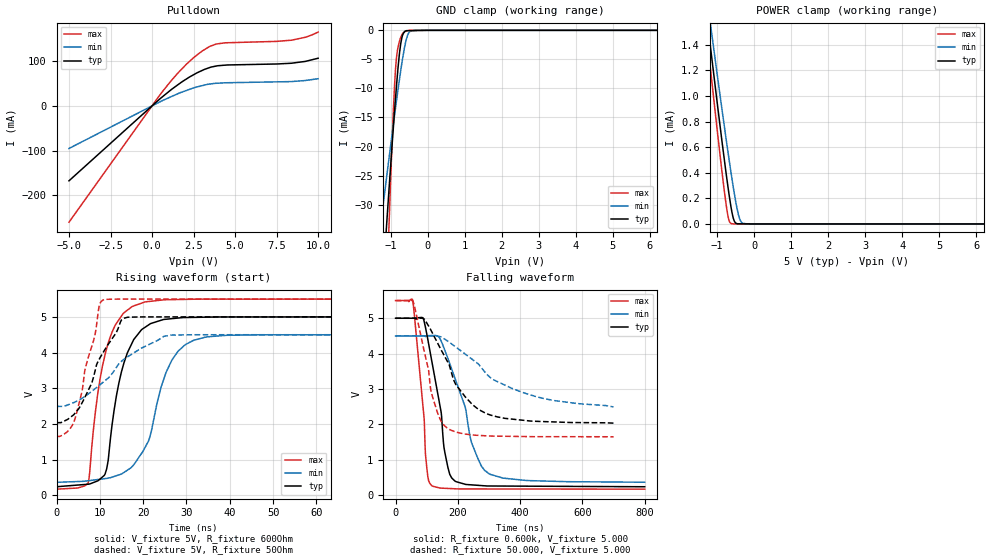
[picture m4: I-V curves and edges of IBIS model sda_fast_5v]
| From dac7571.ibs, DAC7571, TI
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|   SDA_5V IO OPEN DRAIN MODEL
|   5.0V fast mode, freq-3.4M,Rload=600ohm,  Cload = 15pF
[Model]   sda_fast_5v
Model_type   I/O_open_drain
Polarity   Non-Inverting
Enable   Active-Low
Vinl = 1.5
Vinh = 3.5
Vmeas = 2.5
Vref = 5.0
Cref = 15pF
Rref = 600
|   typ   min   max
|   (nom PVT)   (Fast PVT)   (Slow PVT)
|Average
C_comp   5.040e-12   2.855e-12   5.061e-12
|ON state : BUFFER OUTPUT TURNED LOW
|C_comp   6.129e-11   2.855e-11   1.162e-10
|OFF state : BUFFER IN HIGH IMPEDANCE STATE
|C_comp   5.061e-12   5.094e-12   5.040e-12
|Where nom PVT is NOM Process, 5.0V,25C
|   Fast PVT is Strong Process, 5.5V, -40C
|   Slow PVT is Weak Process, 4.5V, 105C
[Model spec]
|   typ   min   max
Vinl   1.5   1.35   1.65
Vinh   3.5   3.15   3.85
[Voltage Range]   5   4.5   5.5
|Junction temperature
[Temperature Range]   25   105   -40
[Pullup Reference]   5   4.5   5.5
[Pulldown Reference]   0   0   0
[Power Clamp Reference]   5   4.5   5.5
[GND Clamp Reference]   0   0   0
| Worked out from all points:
|   slope of the pulldown table from 0 to 0.75 V, typ, clamps not added: 31.1 ohm
|   GND clamp passes 1 mA (typ) near -0.68 V on its own axis
|   POWER clamp passes 1 mA (typ) near -1.02 V on its own axis
|   falling waveform, R_fixture 0.600k, V_fixture 5.000: 20-80 % time 47.7ns typ, 81.4ns min, 28.1ns max; typ from 5 V to 0.238 V
|   rising waveform, V_fixture 5V, R_fixture 600Ohm: 20-80 % time 4.46ns typ, 6.46ns min, 4.34ns max; typ from 0.238 V to 5 V
|   falling waveform, R_fixture 50.000, V_fixture 5.000: 20-80 % time 111ns typ, 204ns min, 55.6ns max; typ from 5 V to 2.04 V
|   rising waveform, V_fixture 5V, R_fixture 50Ohm: 20-80 % time 6.88ns typ, 11.3ns min, 4.33ns max; typ from 2.03 V to 5 V
[Pulldown]
|   Voltage   I(typ)   I(min)   I(max)
-5V       -167.6mA   -95.21mA   -260.1mA
632mV     20.56mA    11.88mA    32.24mA
1.567V    47.51mA    27.48mA    73.88mA
2.073V    60.23mA    34.53mA    93.27mA
3.03V     79.48mA    45.34mA    123mA
3.475V    85.81mA    48.85mA    133mA
3.866V    89.13mA    50.56mA    138.4mA
4.41V     91.14mA    51.64mA    141.1mA
7.49V     93.71mA    53.75mA    144.3mA
8.398V    95.44mA    54.36mA    146.9mA
9.239V    99.6mA     56.83mA    153.6mA
10V       106.6mA    60.8mA     165.1mA
[GND Clamp]
|   Voltage   I(typ)   I(min)   I(max)
-5V       -412.1mA   -229.4mA   -786.8mA
-1.266V   -48.89mA   -33.49mA   -75.73mA
-1.101V   -33mA      -25.04mA   -44.62mA
-1.04V    -27.31mA   -21.99mA   -33.44mA
-924.5mV  -16.82mA   -16.27mA   -14.04mA
-886mV    -13.47mA   -14.41mA   -8.932mA
-847.5mV  -10.29mA   -12.56mA   -5.324mA
-725mV    -2.321mA   -6.967mA   -1.233mA
-575mV    -62.02uA   -1.604mA   -142.6uA
-495.5mV  -53.37uA   -326.8uA   -12.8uA
-324.5mV  -34.76uA   -2.562uA   -8.377uA
10V       0A         0A         0A
[POWER Clamp]
|   Voltage   I(typ)   I(min)   I(max)
-5V       10.92mA    10.1mA     11.74mA
-1.335V   1.762mA    1.9mA      1.632mA
-1.265V   1.591mA    1.747mA    1.443mA
-1.238V   1.526mA    1.688mA    1.371mA
-1.15V    1.313mA    1.498mA    1.136mA
-748.5mV  378.2uA    647.3uA    135.5uA
-688mV    251.5uA    526.5uA    38.06uA
-622mV    128.1uA    396.8uA    2.687uA
-535mV    22.14uA    238.1uA    46.65nA
-428mV    1.278uA    76.93uA    37.34nA
-306.5mV  910.7nA    4.902uA    26.77nA
10V       0A         0A         0A
[Ramp]
R_load = 600
|   typ   min   max
dV/dt_r   2.85718/4.40572e-09   2.48289/6.38671e-09   3.19799/4.32733e-09
dV/dt_f   2.78474/4.60403e-08   0.852531/3.54328e-08   3.19353/2.80374e-08
[Falling Waveform]
R_fixture = 0.600k
V_fixture = 5.000
V_fixture_min = 4.500
V_fixture_max = 5.500
|  time   V(typ)   V(min)   V(max)
0s        5V         4.5V       5.5V
55.1ns    5V         4.5V       5.502V
91.66ns   4.916V     4.5V       2.169V
100.2ns   4.557V     4.498V     786mV
116.1ns   3.799V     4.511V     271.3mV
159.1ns   1.17V      4.073V     194.2mV
192ns     393.3mV    3.272V     181mV
245.1ns   290.7mV    1.458V     176.7mV
302.4ns   259.8mV    597.8mV    176mV
800ns     238.2mV    366mV      170mV
[Rising Waveform]
V_fixture = 5V
V_fixture_min = 4.5V
V_fixture_max = 5.5V
R_fixture = 600Ohm
|   Time   V(typ)   V(min)   V(max)
0s        238mV      361.8mV    170mV
7.308ns   308.7mV    406.2mV    351.7mV
9.414ns   397.8mV    438.6mV    2.753V
11.17ns   586.8mV    465.6mV    3.922V
14.4ns    3.148V     570.1mV    4.919V
17.53ns   4.29V      811.7mV    5.295V
21.26ns   4.775V     1.525V     5.432V
26.6ns    4.95V      3.781V     5.484V
31.64ns   4.987V     4.343V     5.495V
100ns     5V         4.5V       5.5V
[Falling Waveform]
R_fixture = 50.000
V_fixture = 5.000
V_fixture_min = 4.500
V_fixture_max = 5.500
|  time   V(typ)   V(min)   V(max)
0s        5V         4.5V       5.5V
56.25ns   5V         4.5V       5.473V
105.7ns   4.786V     4.501V     3.543V
117.4ns   4.597V     4.501V     2.819V
144.6ns   4.135V     4.477V     2.119V
173.3ns   3.654V     4.319V     1.857V
223ns     2.786V     3.991V     1.727V
300.8ns   2.276V     3.35V      1.673V
461.9ns   2.084V     2.762V     1.653V
700ns     2.036V     2.493V     1.65V
[Rising Waveform]
V_fixture = 5V
V_fixture_min = 4.5V
V_fixture_max = 5.5V
R_fixture = 50Ohm
|   Time   V(typ)   V(min)   V(max)
0s        2.033V     2.492V     1.65V
4.178ns   2.286V     2.606V     2.114V
5.884ns   2.588V     2.717V     2.906V
6.654ns   2.772V     2.778V     3.569V
8.845ns   3.46V      2.981V     4.474V
9.878ns   3.819V     3.083V     5.318V
10.76ns   4.001V     3.169V     5.474V
15.55ns   4.963V     3.812V     5.5V
26.44ns   5V         4.489V     5.5V
100ns     5V         4.5V       5.5V
